FUNCTION "Auto/Cycle ABB" : VOID
TITLE =Auto loader
VERSION : 0.1

BEGIN
NETWORK
TITLE =Ausiliario ciclo singolo ABB
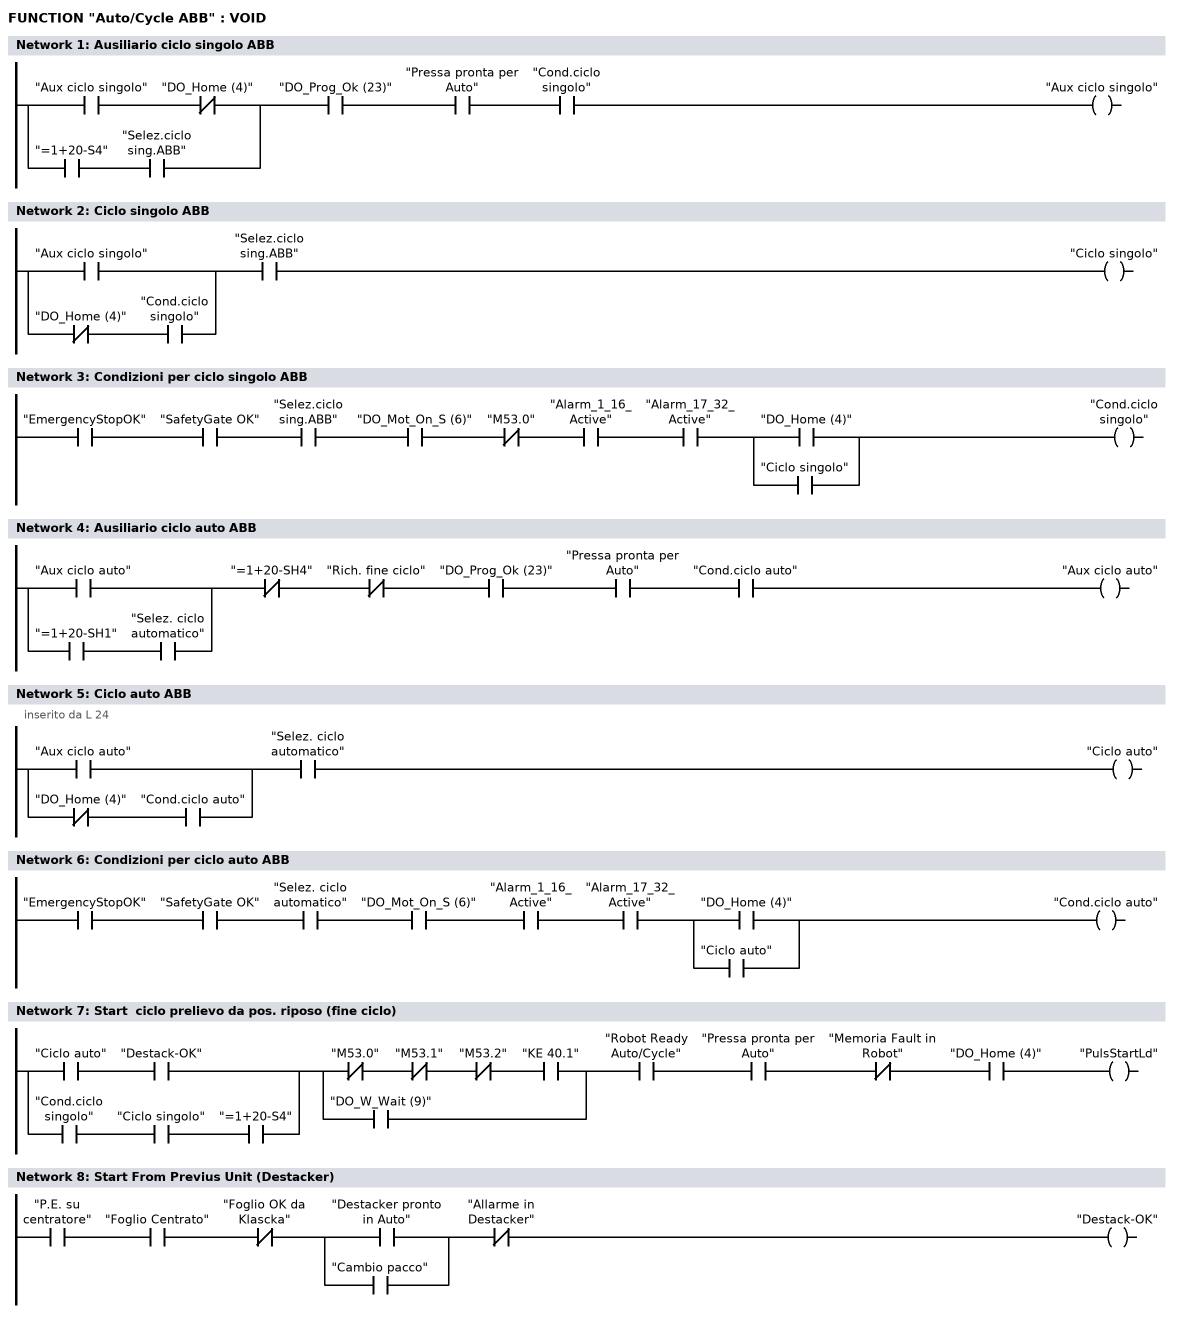
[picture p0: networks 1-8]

      U(    ;
      U     "Aux ciclo singolo";
      UN    "DO_Home (4)";
      O     ;
      U     "=1+20-S4";
      U     "Selez.ciclo sing.ABB";
      )     ;
      U     "DO_Prog_Ok (23)";
      U     "Pressa pronta per Auto";
      U     "Cond.ciclo singolo";
      =     "Aux ciclo singolo";
NETWORK
TITLE =Ciclo singolo ABB

      U(    ;
      O     "Aux ciclo singolo";
      O     ;
      UN    "DO_Home (4)";
      U     "Cond.ciclo singolo";
      )     ;
      U     "Selez.ciclo sing.ABB";
      =     "Ciclo singolo";
NETWORK
TITLE =Condizioni per ciclo singolo ABB

      U     "EmergencyStopOK";
      U     "SafetyGate OK";
      U     "Selez.ciclo sing.ABB";
      U     "DO_Mot_On_S (6)";
      UN    "M53.0";
      U     "Alarm_1_16_Active";
      U     "Alarm_17_32_Active";
      U(    ;
      O     "DO_Home (4)";
      O     "Ciclo singolo";
      )     ;
      =     "Cond.ciclo singolo";
NETWORK
TITLE =Ausiliario ciclo auto ABB

      U(    ;
      O     "Aux ciclo auto";
      O     ;
      U     "=1+20-SH1";
      U     "Selez. ciclo automatico";
      )     ;
      UN    "=1+20-SH4";
      UN    "Rich. fine ciclo";
      U     "DO_Prog_Ok (23)";
      U     "Pressa pronta per Auto";
      U     "Cond.ciclo auto";
      =     "Aux ciclo auto";
NETWORK
TITLE =Ciclo auto ABB
//inserito da L 24
      U(    ;
      O     "Aux ciclo auto";
      O     ;
      UN    "DO_Home (4)";
      U     "Cond.ciclo auto";
      )     ;
      U     "Selez. ciclo automatico";
      =     "Ciclo auto";
NETWORK
TITLE =Condizioni per ciclo auto ABB

      U     "EmergencyStopOK";
      U     "SafetyGate OK";
      U     "Selez. ciclo automatico";
      U     "DO_Mot_On_S (6)";
      U     "Alarm_1_16_Active";
      U     "Alarm_17_32_Active";
      U(    ;
      O     "DO_Home (4)";
      O     "Ciclo auto";
      )     ;
      =     "Cond.ciclo auto";
NETWORK
TITLE =Start  ciclo prelievo da pos. riposo (fine ciclo)

      U(    ;
      U     "Ciclo auto";
      U     "Destack-OK";
      O     ;
      U     "Cond.ciclo singolo";
      U     "Ciclo singolo";
      U     "=1+20-S4";
      )     ;
      U(    ;
      UN    "M53.0";
      UN    "M53.1";
      UN    "M53.2";
      U     "KE 40.1";
      O     "DO_W_Wait (9)";
      )     ;
      U     "Robot Ready Auto/Cycle";
      U     "Pressa pronta per Auto";
      UN    "Memoria Fault in Robot";
      U     "DO_Home (4)";
      =     "PulsStartLd";
NETWORK
TITLE =Start From Previus Unit (Destacker)

      U     "P.E. su centratore";
      U     "Foglio Centrato";
      UN    "Foglio OK da Klascka";
      U(    ;
      O     "Destacker pronto in Auto";
      O     "Cambio pacco";
      )     ;
      UN    "Allarme in Destacker";
      =     "Destack-OK";
END_FUNCTION

